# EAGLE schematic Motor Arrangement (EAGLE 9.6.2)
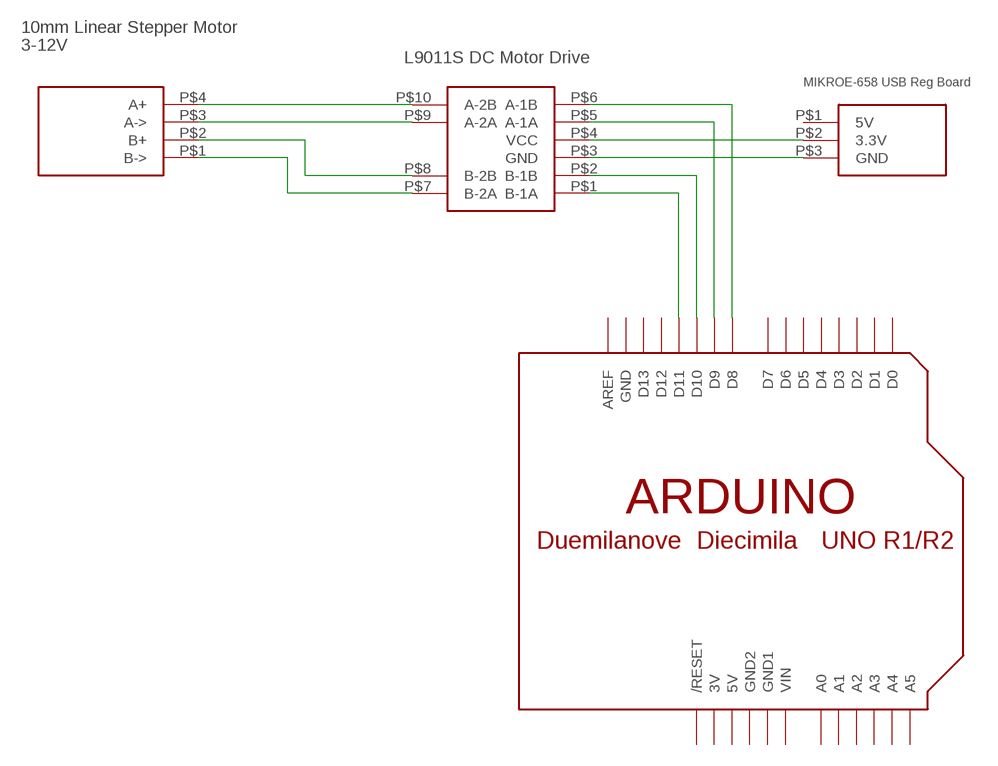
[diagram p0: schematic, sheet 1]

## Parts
U$1  MIKROE-658  [MIKROE-658]
U$2  ARDUINO-NODIM  [ARDUINO-NODIM]
U$3  L9110S  [L9110S]
U$4  10MM-LINEAR-STEPPER  [10MM-LINEAR-STEPPER]

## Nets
N$1: U$1.P$2(3.3V) U$3.P$4(VCC)
N$2: U$1.P$3(GND) U$3.P$3(GND)
N$3: U$3.P$10(A-2B) U$4.P$4(A+)
N$4: U$3.P$9(A-2A) U$4.P$3(A->)
N$5: U$3.P$8(B-2B) U$4.P$2(B+)
N$6: U$3.P$7(B-2A) U$4.P$1(B->)
N$7: U$2.D8 U$3.P$6(A-1B)
N$8: U$2.D9 U$3.P$5(A-1A)
N$9: U$2.D10 U$3.P$2(B-1B)
N$10: U$2.D11 U$3.P$1(B-1A)
Unconnected: U$1.P$1(5V) U$2.A0 U$2.A1 U$2.A2 U$2.A3 U$2.A4 U$2.A5 U$2.AREF U$2.D0 U$2.D1 U$2.D2 U$2.D3 U$2.D4 U$2.D5 U$2.D6 U$2.D7 U$2.D12 U$2.D13 U$2.RESET(/RESET)

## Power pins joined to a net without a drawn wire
3V: U$2.3V
5V: U$2.5V
GND: U$2.GND
GND1: U$2.GND1
GND2: U$2.GND2
VIN: U$2.VIN

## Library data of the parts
U$1 = MotorArrangement:MIKROE-658
U$2 = adafruit:ARDUINO: Arduino Diecimila/Duemilanove Make a shield with ease, this package has all the named pins as well as the two mounting drill holes and an outline of the USB and DC power connector. The outline is on the DIMENSION layer, so if your board house uses it they will cut the outline to match.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
U$3 = MotorArrangement:L9110S
U$4 = MotorArrangement:10MM-LINEAR-STEPPER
